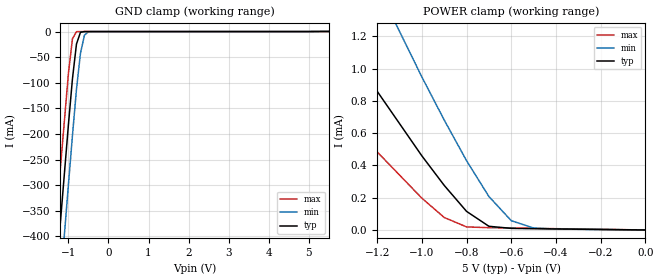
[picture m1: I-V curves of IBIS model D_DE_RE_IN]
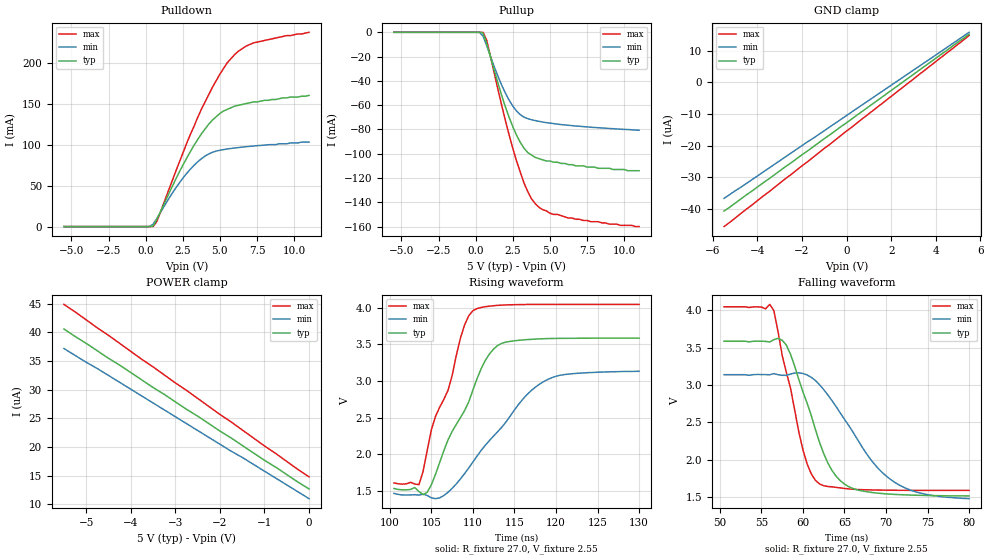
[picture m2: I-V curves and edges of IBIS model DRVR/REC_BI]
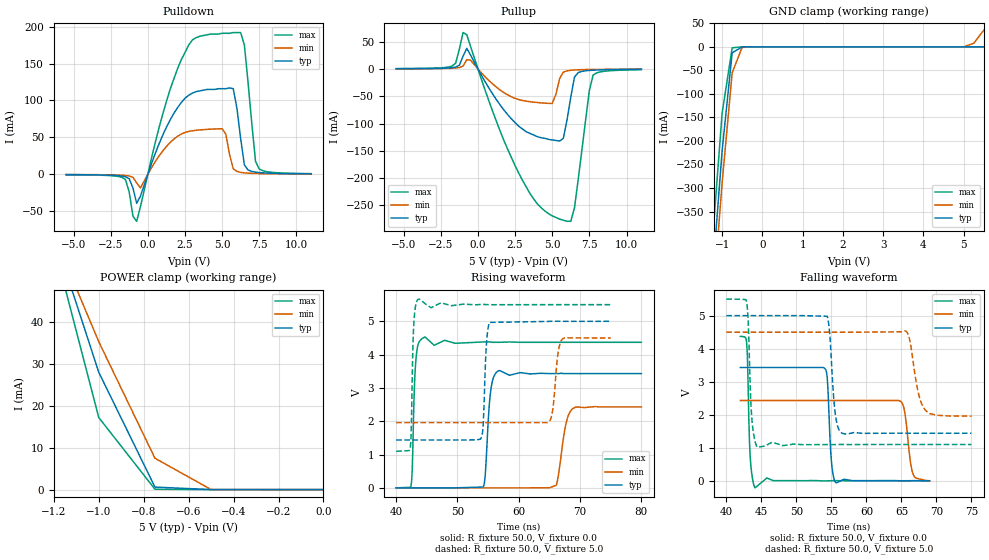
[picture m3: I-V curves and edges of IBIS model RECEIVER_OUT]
|   Texas Instruments Incorporated
|   Data Transmissions Products
|   IBIS Model for SN65HVD485
|   8D SOIC Package
[IBIS Ver]   3.2
[Comment char]   |_char
[File name]   hvd485e.ibs
[File Rev]   1.0
[Date]   8December03
[Source]   File originated at Texas Instruments Incorporated.
   Data Transmission Products Group.
[Notes]
[Disclaimer]
(C) Copyright Texas Instruments Incorporated 2002
   All rights reserved
  Texas Instruments Incorporated hereby grants the user of this IBIS
model a non-exclusive, nontransferable license to use this IBIS model
under the following terms.  Before using this IBIS model, the user
should read this license.  If the user does not accept these terms,
the IBIS model should be returned to Texas Instruments within 30 days.
  The user is granted this license only to use the IBIS model and
is not granted rights to sell, load, rent, lease or license the IBIS
model in whole or in part, or in modified form to anyone other than
user.  User may modify the IBIS model to suit its specific applications
but rights to derivative works and such modifications shall belong to
Texas Instruments.
  This IBIS model is provided on an "AS IS" basis and Texas Instruments
makes absolutely no warranty with respect to the information contained
herein.  TEXAS INSTRUMENTS DISCLAIMS AND CUSTOMER WAIVES ALL WARRANTIES,
EXPRESS OR IMPLIED, INCLUDING WARRANTIES OF MERCHANTABILITY OR FITNESS
FOR A PARTICULAR PURPOSE. The entire risk as to quality and performance
is with the Customer. ACCORDINGLY, IN NO EVENT SHALL THE COMPANY BE LIABLE
FOR ANY DAMAGES, WHETHER IN CONTRACT OR TORT,INCLUDING ANY LOST PROFITS
OR OTHER INCIDENTAL, CONSEQUENTIAL, EXEMPLARY, OR PUNITIVE DAMAGES ARISING
OUT OF THE USE OR APPLICATION OF THE IBIS model provided in this package.
Further, Texas Instruments reserves the right to discontinue or make changes
without notice to any product herein to improve reliability, function, or
design. Texas Instruments does not convey any license under patent rights
or any other intellectual property rights, including those of third parties.
Contact Texas Instruments at ATTN:DATA TRANSMISSIONS
[Copyright]   Copyright 2002, Texas Instruments, All Rights Reserved
[Component]   HVD485ED
[Manufacturer]  Texas Instruments Incorporated
[Package]
|   typ   min   max
R_pkg   0.055   0.034   0.067
L_pkg   1.795nH   1.699nH   1.914nH
C_pkg   0.299pF   0.278pF   0.311pF
[Pin]   signal_name   model_name   R_pin   L_pin   C_pin
1   R   RECEIVER_OUT   0.067   1.914n   0.278p
2   RE   D_DE_RE_IN   0.062   1.816n   0.301p
3   DE   D_DE_RE_IN   0.053   1.699n   0.298p
4   D   D_DE_RE_IN   0.067   1.907n   0.278p
5   GND   GND   0.034   1.704n   0.311p
6   A   DRVR/REC_BI   0.061   1.808n   0.310p
7   B   DRVR/REC_BI   0.062   1.817n   0.302p
8   VCC   POWER   0.034   1.716n   0.311p
[Diff_pin]   inv_pin   vdiff   tdelay_typ   tdelay_min   tdelay_max
| The 'A' pin is Diff_pin and the 'B' pin is the inv_pin
6   7   0.200   0 0 0
| Models and submodels in the file (3): D_DE_RE_IN (Input), DRVR/REC_BI (I/O), RECEIVER_OUT (3-state)
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|   Driver Input / Driver Enable / Receiver Enable Model
[Model]   D_DE_RE_IN
Model_type   Input
|Signals   D,DE,RE
Vinh = 2.0
Vinl = 0.8
|   typ   min   max
C_comp   8.8pF   7.0pF   10.6pF
|   typ   min   max
[Temperature Range]   27   -40   85
[Voltage range]   5.0V   4.5V   5.5V
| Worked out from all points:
|   GND clamp passes 1 mA (typ) near -0.67 V on its own axis
[GND_clamp]
|   Voltage   I(typ)   I(min)   I(max)
-5.5V     -4.24A     -4.45A     -4.05A
-1.5V     -656mA     -783mA     -541mA
-1V       -181mA     -298mA     -81mA
-900mV    -92.1mA    -203mA     -14mA
-800mV    -24.4mA    -113mA     -243uA
-700mV    -1.47mA    -42.5mA    -35.7uA
-600mV    -60.2uA    -6.95mA    -34.3uA
-500mV    -28.2uA    -440uA     -34.2uA
5.5V      8.03uA     948uA      13.6pA
[Power_clamp]
| Note that the[POWER_clamp]voltage table is referenced to Vcc
| and is calculated using Vtable=Vcc - Vmeasured.
|   Voltage   I(typ)   I(min)   I(max)
-5.5V     9.87mA     14.2mA     6.98mA
-2V       2.49mA     3.81mA     1.66mA
-1.5V     1.46mA     2.36mA     914uA
-1V       459uA      948uA      197uA
-900mV    276uA      681uA      77.3uA
-800mV    115uA      429uA      18.9uA
-700mV    22.7uA     207uA      14.1uA
-600mV    9.99uA     57.3uA     12uA
-500mV    8.03uA     12.1uA     9.98uA
-400mV    6.37uA     5.86uA     7.93uA
0V        0A         0A         0A
|   Driver Output / Receiver Input Model
[Model]   DRVR/REC_BI
Model_type   I/O
| Signals   A,B
Vinl = 0.9V
Vinh = 2.8V
Vmeas = 1.7V   |Reference voltage for timing measurements
Cref = 50pF   |Timing specification test load capacitance value
Rref = 54   |Note: 54 Ohm load; single-ended configuration
|   Timing specification test load voltage
| variable   typ   min   max
C_comp   13.3pF   10.7pF   16.0pF
|   typ   min   max
[Temperature Range]   25.0   -40   85
[Voltage range]   5.0V   4.5V   5.5V
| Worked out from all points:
|   slope of the pulldown table from 0 to 0.75 V, typ, clamps not added: 89.2 ohm
|   slope of the pullup table from 0 to 0.75 V, typ, clamps not added: 79.1 ohm
|   rising waveform, R_fixture 27.0, V_fixture 2.55: 20-80 % time 4.85ns typ, 6.98ns min, 3.87ns max; typ from 1.53 V to 3.59 V
|   falling waveform, R_fixture 27.0, V_fixture 2.55: 20-80 % time 3.91ns typ, 6.34ns min, 2.88ns max; typ from 3.59 V to 1.51 V
[Pulldown]
|   Voltage   I(typ)   I(min)   I(max)
-5.5V     -28.1nA    -33.7nA    -24.1nA
250mV     123nA      21.1uA     -28.1nA
500mV     666uA      2.79mA     13.9uA
750mV     8.41mA     9.81mA     6.1mA
2.25V     65.9mA     52.8mA     77.8mA
3.25V     98.9mA     74.6mA     122mA
3.75V     113mA      82.7mA     143mA
4.5V      130mA      90.6mA     170mA
5.5V      143mA      94.7mA     200mA
6.25V     148mA      96.4mA     214mA
7.25V     152mA      98.2mA     224mA
11V       160mA      103mA      237mA
[Pullup]
|   Voltage   I(typ)   I(min)   I(max)
| Note that the[Pullup]voltage table is referenced to Vcc
| and is calculated using Vtable=Vcc - Vmeasured.
-5.5V     22.3nA     22.5nA     16.8nA
250mV     -132nA     -21.2uA    18.4nA
500mV     -700uA     -3.14mA    -13.9uA
750mV     -9.48mA    -11.3mA    -6.85mA
1.75V     -52mA      -43.5mA    -60.1mA
2.5V      -77.8mA    -60.8mA    -95.6mA
3.25V     -95.4mA    -69.9mA    -124mA
3.75V     -101mA     -72mA      -137mA
4V        -103mA     -72.7mA    -141mA
5V        -106mA     -74.8mA    -149mA
6.25V     -109mA     -76.6mA    -153mA
11V       -114mA     -80.7mA    -160mA
[GND_clamp]
|   Voltage  I(typ)   I(min)   I(max)
| Outputs in High Impedance (off)
-5.5V     -40.7uA    -36.7uA    -45.6uA
-1.75V    -21.7uA    -18.8uA    -25.1uA
-1.5V     -20.4uA    -17.7uA    -23.7uA
5.5V      15.2uA     15.8uA     14.8uA
[POWER_clamp]
|   Voltage  I(typ)   I(min)   I(max)
| Note that the [POWER_clamp] voltage table is referenced to Vcc
| and is calculated using Vtable = Vcc - Vmeasured.
| Outputs in Tri-state.
-5.5V     40.6uA     37.2uA     44.9uA
-4.75V    36.8uA     33.7uA     40.8uA
-1V       17.7uA     15.8uA     20.2uA
0V        12.7uA     11uA       14.8uA
[Ramp]
|   typ   min   max
dV/dt_r   1.23V/4.8ns   1.00V/7.0ns   1.46V/3.9ns
dV/dt_f   1.24V/3.9ns   1.00V/6.3ns   1.47V/2.9ns
R_load = 27ohm | Note: The measurement is on a single-ended configuration
|   with 54ohm line-to-line.
[Rising Waveform]
R_fixture = 27.0
V_fixture = 2.55
V_fixture_min = 2.276
V_fixture_max = 2.843
C_fixture = 0p
L_fixture = 0n
|   V(typ)   V(min)  V(max)
100.5ns   1.531V     1.464V     1.607V
103.5ns   1.49V      1.441V     1.583V
105ns     1.582V     1.404V     2.334V
107ns     2.195V     1.479V     2.871V
109ns     2.596V     1.735V     3.768V
110ns     2.877V     1.893V     3.96V
111.5ns   3.283V     2.123V     4.016V
113ns     3.487V     2.31V      4.034V
118.5ns   3.578V     2.991V     4.047V
130ns     3.586V     3.133V     4.047V
[Falling Waveform]
R_fixture = 27.0
V_fixture = 2.55
V_fixture_min = 2.276
V_fixture_max = 2.843
C_fixture = 0p
L_fixture = 0n
|   V(typ)   V(min)  V(max)
50.5ns    3.587V     3.139V     4.048V
56.5ns    3.608V     3.153V     3.997V
58ns      3.535V     3.13V      3.17V
60ns      2.907V     3.155V     2.131V
61ns      2.592V     3.104V     1.811V
62ns      2.231V     3.004V     1.676V
63.5ns    1.856V     2.791V     1.637V
65ns      1.674V     2.542V     1.616V
70.5ns    1.54V      1.74V      1.592V
80ns      1.515V     1.479V     1.59V
|   Receiver Output Model
[Model]   RECEIVER_OUT
Model_type   3-state
| Signals   R
Vmeas = 2.2V   |Reference voltage for timing measurements
Cref = 15pF   |Timing specification test load capacitance value
Vref = 0   |Timing specification test load voltage; GND
| variable   typ   min   max
C_comp   10.2pF   8.2pF   12.2pF
|   typ   min   max
[Temperature Range]   25.0   -40   85
[Voltage range]   5.0V   4.5V   5.5V
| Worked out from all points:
|   slope of the pulldown table from 0 to 0.75 V, typ, clamps not added: 18.3 ohm
|   slope of the pullup table from 0 to 0.75 V, typ, clamps not added: 21.1 ohm
|   GND clamp passes 1 mA (typ) near -0.52 V on its own axis
|   POWER clamp passes 1 mA (typ) near -0.75 V on its own axis
|   rising waveform, R_fixture 50.0, V_fixture 0.0: 20-80 % time 683ps typ, 1.18ns min, 422ps max; typ from 0 V to 3.43 V
|   falling waveform, R_fixture 50.0, V_fixture 0.0: 20-80 % time 455ps typ, 788ps min, 333ps max; typ from 3.43 V to -0.001 V
|   rising waveform, R_fixture 50.0, V_fixture 5.0: 20-80 % time 457ps typ, 749ps min, 311ps max; typ from 1.44 V to 5 V
|   falling waveform, R_fixture 50.0, V_fixture 5.0: 20-80 % time 666ps typ, 1.24ns min, 447ps max; typ from 5 V to 1.44 V
[Pulldown]
|   Voltage   I(typ)   I(min)   I(max)
-5.5V     -420uA     -260uA     -560uA
-1.5V     -3.32mA    -1.54mA    -7.13mA
-750mV    -39.1mA    -11.6mA    -63.6mA
-500mV    -29.8mA    -18.4mA    -44.2mA
1.25V     63.7mA     37.6mA     98.5mA
2.75V     107mA      58.1mA     175mA
5V        116mA      61.8mA     191mA
5.75V     116mA      7.56mA     192mA
6.5V      12.8mA     2mA        175mA
7.25V     2.97mA     1.15mA     17.6mA
7.5V      2.39mA     1.01mA     7.26mA
11V       641uA      367uA      950uA
[Pullup]
|   Voltage   I(typ)   I(min)   I(max)
| Note that the[Pullup]voltage table is referenced to Vcc
| and is calculated using Vtable=Vcc - Vmeasured.
-5.5V     388uA      251uA      620uA
-1.75V    2.29mA     1.22mA     5.08mA
-1V       23.4mA     5.37mA     66.6mA
-750mV    37.7mA     17mA       62.6mA
3V        -110mA     -57.7mA    -204mA
5V        -130mA     -63.2mA    -269mA
5.75V     -127mA     -5.86mA    -277mA
6V        -92.7mA    -3.45mA    -279mA
6.5V      -14.7mA    -1.91mA    -254mA
7.5V      -2.71mA    -990uA     -39.3mA
7.75V     -2.27mA    -890uA     -11.4mA
11V       -190uA     -90uA      -1.5mA
[GND_clamp]
|   Voltage   I(typ)   I(min)   I(max)
| Outputs in High Impedance (off)
-5.5V     -5.07A     -5.05A     -5.12A
-1.25V    -500mA     -565mA     -423mA
-1V       -221mA     -289mA     -141mA
-750mV    -12.7mA    -55mA      -2.02mA
-500mV    -8.18uA    -416uA     -41.3uA
5V        65.5pA     16.7uA     61.8pA
5.25V     77.3pA     7.48mA     69.1pA
5.5V      47nA       35.3mA     74.6pA
[POWER_clamp]
|   Voltage  I(typ)   I(min)   I(max)
| Note that the [POWER_clamp] voltage table is referenced to Vcc
| and is calculated using Vtable = Vcc - Vmeasured.
| Outputs in Tri-state.
-5.5V     830mA      648mA      1.05A
-1.25V    69.2mA     67.2mA     68.8mA
-1V       28mA       35.3mA     17.2mA
-750mV    606uA      7.48mA     88.4uA
-500mV    47nA       16.7uA     12.1nA
0V        65.5pA     144pA      74.6pA
[Ramp]
|   typ   min   max
dV/dt_r   2.14V/569ns   1.53V/1170ps   2.64V/311ps
dV/dt_f   2.14V/561ps   1.53V/1240ps   2.64V/333ps
R_load = 50
[Rising Waveform]
R_fixture = 50.0
V_fixture = 0.0
C_fixture = 0p
L_fixture = 0n
|   V(typ)   V(min)   V(max)
40ns      3.04uV     3uV        293uV
42.4ns    2.06uV     4.91uV     46.5mV
43.2ns    14.1uV     4.33uV     3.81V
44.2ns    36.2uV     3.07uV     4.48V
54.2ns    25.8mV     13.1uV     4.38V
55.4ns    2.89V      16.1uV     4.38V
56.6ns    3.51V      19.5uV     4.37V
66.1ns    3.43V      75.6mV     4.37V
68.8ns    3.43V      2.38V      4.37V
80ns      3.43V      2.43V      4.37V
[Falling Waveform]
R_fixture = 50.0
V_fixture = 0.0
C_fixture = 0p
L_fixture = 0n
|   V(typ)   V(min)   V(max)
42ns      3.43V      2.43V      4.37V
42.9ns    3.43V      2.43V      4.18V
43.4ns    3.43V      2.43V      744mV
44.1ns    3.43V      2.43V      -216mV
54ns      3.41V      2.43V      -4.55mV
55ns      593mV      2.43V      498uV
55.6ns    -49.7mV    2.43V      2.48mV
64.6ns    -98.1uV    2.43V      -31.8uV
66.7ns    1.11mV     184mV      -22uV
69ns      -525uV     -9.82mV    18.2uV
[Rising Waveform]
R_fixture = 50.0
V_fixture = 5.0
V_fixture_min = 4.5
V_fixture_max = 5.5
C_fixture = 0p
L_fixture = 0n
|   V(typ)   V(min)  V(max)
40ns      1.438V     1.957V     1.097V
42.3ns    1.438V     1.957V     1.202V
42.8ns    1.438V     1.957V     4.656V
43.5ns    1.438V     1.957V     5.651V
53.8ns    1.481V     1.957V     5.505V
54.2ns    1.918V     1.957V     5.506V
55.2ns    4.967V     1.957V     5.498V
64.8ns    4.997V     1.965V     5.5V
67ns      5V         4.442V     5.5V
75ns      5V         4.5V       5.5V
[Falling Waveform]
R_fixture = 50.0
V_fixture = 5.0
V_fixture_min = 4.5
V_fixture_max = 5.5
C_fixture = 0p
L_fixture = 0n
|   V(typ)   V(min)  V(max)
40ns      5V         4.5V       5.5V
42.9ns    5V         4.5V       5.415V
43.6ns    5V         4.5V       1.989V
44.4ns    5V         4.5V       1.017V
54.4ns    4.982V     4.5V       1.095V
55.5ns    2.119V     4.5V       1.096V
56.5ns    1.445V     4.5V       1.098V
65.6ns    1.439V     4.533V     1.097V
68.4ns    1.438V     2.141V     1.097V
75ns      1.438V     1.957V     1.097V
